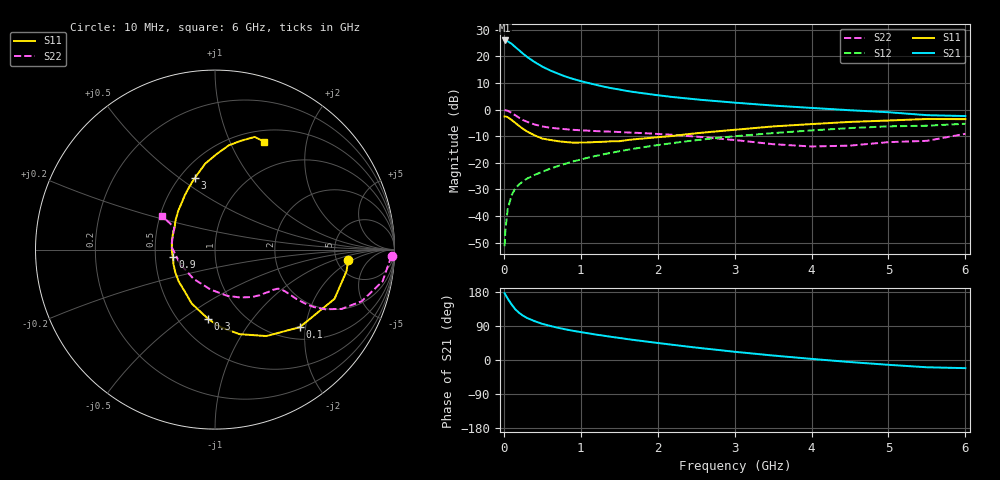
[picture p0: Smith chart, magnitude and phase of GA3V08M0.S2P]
! Infineon Technologies  Discrete & RF Semiconductors
! BF775
! Si NPN RF Bipolar Junction Transistor in SOT23
! VCE = 3 V  IC = 8 mA
! Common Emitter S-Parameters:  May  1996
# GHz  S  MA  R  50
!  f  S11  S21  S12  S22
! GHz  MAG  ANG  MAG  ANG  MAG  ANG  MAG  ANG
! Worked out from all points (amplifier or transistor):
!   36 points, 10 MHz to 6 GHz, reference 50 ohm
!   highest |S21| = 26.0 dB at 10 MHz (marker M1)
!   |S21| within 3 dB of that: start of sweep to 170.2 MHz
!   unconditionally stable (mu >= 1): 634.5 MHz to 3.389 GHz
!   at 250 MHz: K = 0.63, MSG = 24.0 dB, |S12| = -27.0 dB
!   at 1.4 GHz: K = 1.12, MAG = 10.0 dB, |S12| = -16.2 dB
!   at 6 GHz: K = 0.96, MSG = 1.4 dB, |S12| = -5.3 dB
!   S11 on the Smith chart (normalised r, x): 10 MHz: 6.33, -1.68; 100 MHz: 1.27, -1.86; 300 MHz: 0.69, -0.63; 900 MHz: 0.62, -0.05; 3 GHz: 0.59, +0.58; 6 GHz: 0.63, +1.35
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0.01  0.7431 -4.6  19.94 176.3  0.0027 84.2  0.9855 -2.1
0.02  0.743 -9.2  19.63 172.4  0.0054 85.0  0.9717 -4.4
0.05  0.7201 -22.4  19.22 162.0  0.0134 77.8  0.9505 -10.7
0.1  0.6401 -42.5  17.32 146.7  0.0244 71.1  0.8665 -19.4
0.15  0.5602 -59.3  14.94 133.6  0.0333 64.8  0.779 -25.1
0.2  0.4907 -73.8  12.99 124.2  0.0393 62.0  0.6989 -28.4
0.25  0.4338 -85.7  11.22 116.8  0.0449 60.2  0.6351 -30.2
0.3  0.3887 -95.5  9.819 111.1  0.0502 59.7  0.5899 -30.9
0.4  0.3274 -113.4  7.836 102.5  0.059 59.9  0.5247 -31.2
0.5  0.2852 -127.1  6.424 95.4  0.0675 60.4  0.4821 -30.9
0.6  0.2688 -139.1  5.467 90.0  0.0772 61.1  0.4569 -30.8
0.7  0.2548 -150.2  4.763 85.2  0.0862 61.6  0.4405 -30.9
0.9  0.2388 -170.0  3.768 77.0  0.1059 62.2  0.4161 -31.6
1.1  0.2412 175.4  3.158 70.3  0.1253 62.1  0.4009 -33.6
1.3  0.2478 162.9  2.701 64.1  0.1448 61.1  0.3886 -35.8
1.6  0.2664 146.6  2.241 55.3  0.1746 59.0  0.372 -40.3
2.2  0.3196 125.5  1.719 40.0  0.235 53.7  0.3351 -52.0
3  0.4166 105.4  1.351 21.7  0.3151 44.6  0.2676 -74.8
3.5  0.4821 96.5  1.19 11.8  0.3612 38.3  0.2236 -96.5
4.5  0.5864 82.4  0.972 -5.4  0.4484 25.1  0.21 -157.9
5.5  0.6656 70.6  0.785 -19.2  0.4975 10.4  0.2583 151.5
6  0.6608 65.7  0.755 -21.5  0.5416 6.3  0.3504 147.5
